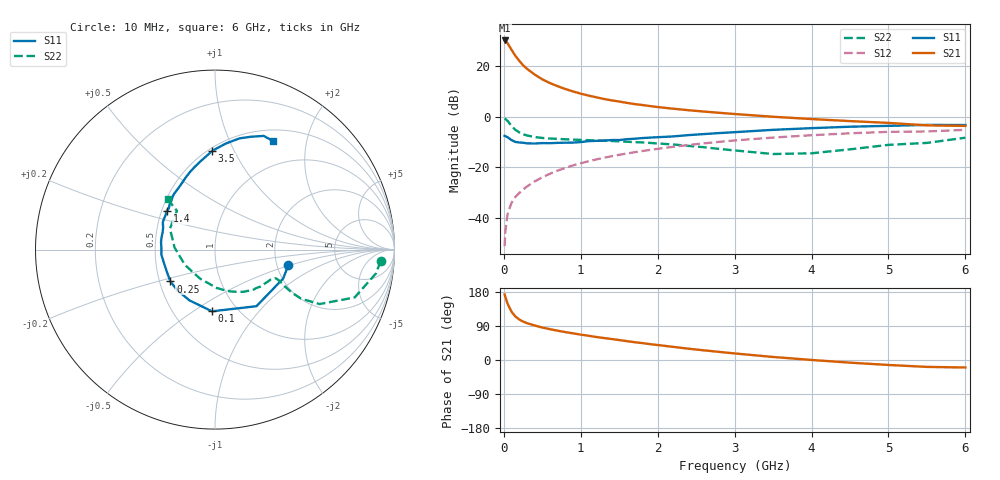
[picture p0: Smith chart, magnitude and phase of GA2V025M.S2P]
! Infineon Technologies  Discrete & RF Semiconductors
! BF775
! Si NPN RF Bipolar Junction Transistor in SOT23
! VCE = 2 V  IC = 25 mA
! Common Emitter S-Parameters:  May  1996
# GHz  S  MA  R  50
!  f  S11  S21  S12  S22
! GHz  MAG  ANG  MAG  ANG  MAG  ANG  MAG  ANG
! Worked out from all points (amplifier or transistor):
!   36 points, 10 MHz to 6 GHz, reference 50 ohm
!   highest |S21| = 30.3 dB at 10 MHz (marker M1)
!   |S21| within 3 dB of that: start of sweep to 86.04 MHz
!   unconditionally stable (mu >= 1): 240.5 MHz to end of sweep
!   at 250 MHz: K = 1.02, MAG = 23.9 dB, |S12| = -28.9 dB
!   at 1.4 GHz: K = 1.19, MAG = 8.4 dB, |S12| = -15.7 dB
!   at 6 GHz: K = 1.03, MAG = -0.3 dB, |S12| = -5.2 dB
!   S11 on the Smith chart (normalised r, x): 10 MHz: 2.31, -0.49; 100 MHz: 0.77, -0.60; 250 MHz: 0.57, -0.22; 1.4 GHz: 0.53, +0.26; 3.5 GHz: 0.52, +0.83; 6 GHz: 0.64, +1.47
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0.01  0.4178 -12.0  32.7 172.9  0.0027 86.3  0.9251 -4.0
0.02  0.4125 -23.0  32.11 165.8  0.0054 81.0  0.9067 -8.4
0.05  0.3909 -53.8  28.54 148.0  0.012 73.3  0.8226 -18.9
0.1  0.3442 -92.8  21.34 127.4  0.0196 66.3  0.6571 -27.5
0.15  0.3167 -116.6  16.24 114.8  0.0256 64.3  0.5512 -29.7
0.2  0.3089 -132.7  12.93 107.0  0.0305 66.0  0.4898 -29.2
0.25  0.3053 -144.4  10.55 101.4  0.0359 66.9  0.4493 -28.1
0.3  0.2967 -152.9  8.975 97.3  0.0412 68.7  0.4256 -27.2
0.4  0.2942 -165.7  6.895 91.1  0.0519 69.9  0.3964 -25.8
0.5  0.2999 -174.6  5.53 85.7  0.0628 71.0  0.3795 -25.3
0.6  0.2987 178.4  4.654 81.3  0.074 70.9  0.3702 -25.5
0.8  0.3055 167.3  3.552 73.6  0.0967 70.1  0.3572 -27.2
0.9  0.3073 161.7  3.178 70.3  0.1084 69.6  0.3514 -28.4
1.1  0.3279 152.5  2.635 64.0  0.1308 68.0  0.343 -31.7
1.4  0.3449 141.1  2.115 55.4  0.1643 65.0  0.3304 -37.1
1.7  0.3664 131.4  1.787 47.0  0.1977 61.6  0.3133 -43.4
2.2  0.4069 118.2  1.446 34.7  0.2533 55.3  0.2819 -56.6
2.8  0.4743 103.8  1.198 21.4  0.318 47.3  0.2299 -77.8
3.5  0.5505 91.6  1 8.0  0.3866 37.1  0.1821 -117.2
4.5  0.6344 77.6  0.82 -7.0  0.47 22.7  0.2257 177.0
5.5  0.6891 66.8  0.675 -18.2  0.5109 7.5  0.3027 134.5
6  0.6857 61.9  0.658 -19.8  0.5505 3.3  0.3842 133.2
